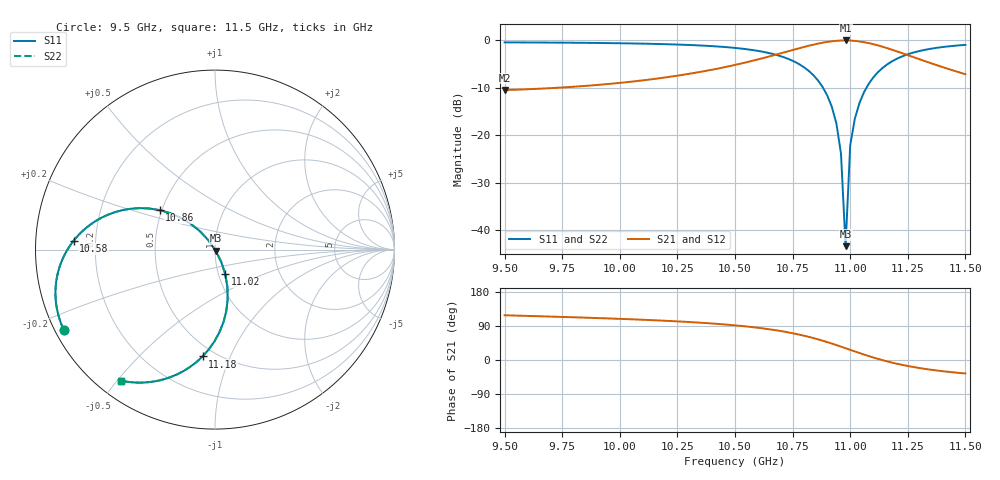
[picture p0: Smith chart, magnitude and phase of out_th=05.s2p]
!freq-unit param-type data-format keyword impedance-ohms
# GHZ  S  MA  R  50
!Freq  MagS11 AngS11 MagS21  AngS21 MagS12 AngS12
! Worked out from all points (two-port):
!   101 points, 9.5 GHz to 11.5 GHz, reference 50 ohm
!   highest |S21| = 0.00 dB at 10.98 GHz (marker M1); lowest = -10.5 dB at 9.5 GHz (marker M2)
!   |S21| within 3 dB of the highest: 10.68 GHz to 11.24 GHz (566.7 MHz wide, 5.17 % of centre)
!   lowest |S11| = -43.4 dB at 10.98 GHz (marker M3), VSWR 1.01, Z = 50.3 - j0.581 ohm
!   |S11| at or under -10 dB: 10.88 GHz to 11.07 GHz (188.4 MHz wide, 1.72 % of centre)
!   |S22| runs from -43.4 to -0.4 dB; largest |S21 - S12| = 0
!   S11 on the Smith chart (normalised r, x): 9.5 GHz: 0.02, -0.25; 10.58 GHz: 0.12, +0.03; 10.86 GHz: 0.49, +0.25; 11.02 GHz: 1.08, -0.30; 11.18 GHz: 0.43, -0.79; 11.5 GHz: 0.07, -0.51
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9.5  0.9541 -151.9  0.2996 118.1  0.2996 118.1  0.9541 -151.9
9.84  0.944 -158.1  0.33 111.9  0.33 111.9  0.944 -158.1
10.18  0.9159 -166.0  0.4015 104.0  0.4015 104.0  0.9159 -166.0
10.5  0.834 -178.6  0.5518 91.4  0.5518 91.4  0.834 -178.6
10.58  0.7897 176.5  0.6135 86.5  0.6135 86.5  0.7897 176.5
10.72  0.6545 164.1  0.756 74.1  0.756 74.1  0.6545 164.1
10.78  0.5591 156.8  0.8291 66.8  0.8291 66.8  0.5591 156.8
10.84  0.4305 147.9  0.9026 57.9  0.9026 57.9  0.4305 147.9
10.86  0.3792 144.5  0.9253 54.5  0.9253 54.5  0.3792 144.5
10.9  0.2638 137.3  0.9646 47.3  0.9646 47.3  0.2638 137.3
10.92  0.2002 133.4  0.9798 43.4  0.9798 43.4  0.2002 133.4
10.94  0.1334 129.4  0.9911 39.4  0.9911 39.4  0.1334 129.4
10.96  0.06411 125.3  0.9979 35.3  0.9979 35.3  0.06411 125.3
10.98  0.006738 -58.9  1 31.1  1 31.1  0.006738 -58.9
11  0.07809 -63.2  0.9969 26.8  0.9969 26.8  0.07809 -63.2
11.02  0.1488 -67.4  0.9889 22.6  0.9889 22.6  0.1488 -67.4
11.04  0.2179 -71.5  0.976 18.5  0.976 18.5  0.2179 -71.5
11.08  0.3475 -79.5  0.9377 10.5  0.9377 10.5  0.3475 -79.5
11.12  0.4614 -86.9  0.8872 3.1  0.8872 3.1  0.4614 -86.9
11.18  0.5992 -96.6  0.8006 -6.6  0.8006 -6.6  0.5992 -96.6
11.3  0.7731 -111.2  0.6343 -21.2  0.6343 -21.2  0.7731 -111.2
11.5  0.8978 -125.5  0.4404 -35.5  0.4404 -35.5  0.8978 -125.5
